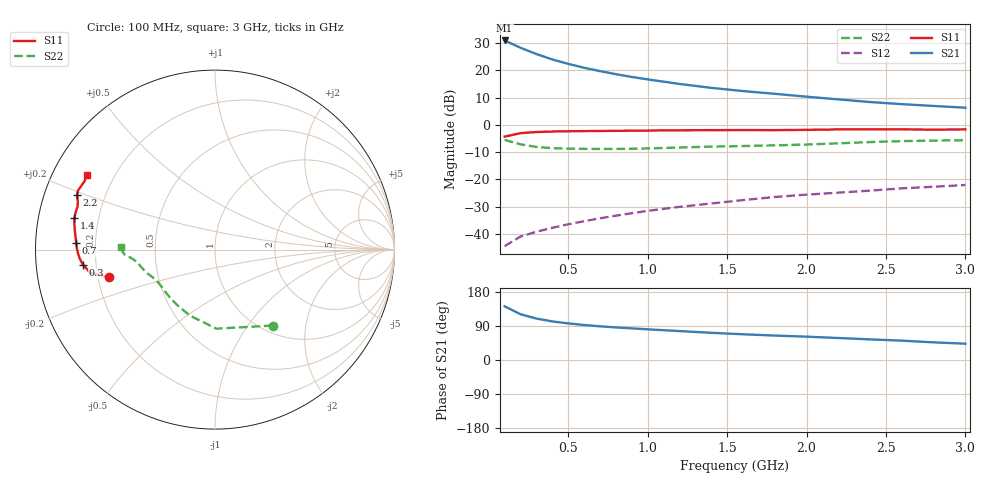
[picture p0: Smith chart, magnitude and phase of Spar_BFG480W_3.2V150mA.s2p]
! Filename: 3_2150BFG480.001
! Title: BFG480W
! Bias: Vce=3.2V; Ic=150mA
! Company: NXP Semiconductors NL
! User: Quality&Reliability T&D
! Measure time: 10 Nov 1999 / 11:58:59
#  MHz  S  MA  R 50
! Freq  S11  S21  S12  S22  :
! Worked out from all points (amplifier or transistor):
!   20 points, 100 MHz to 3 GHz, reference 50 ohm
!   highest |S21| = 30.9 dB at 100 MHz (marker M1)
!   |S21| within 3 dB of that: start of sweep to 213.9 MHz
!   unconditionally stable (mu >= 1): start of sweep to 121.3 MHz; 303.4 MHz to end of sweep
!   at 400 MHz: K = 1.07, MAG = 29.3 dB, |S12| = -37.7 dB
!   at 1.2 GHz: K = 1.20, MAG = 19.8 dB, |S12| = -30.0 dB
!   at 3 GHz: K = 1.16, MAG = 11.8 dB, |S12| = -22.0 dB
!   S11 on the Smith chart (normalised r, x): 100 MHz: 0.25, -0.12; 300 MHz: 0.15, -0.06; 700 MHz: 0.13, +0.02; 1.4 GHz: 0.11, +0.11; 2.2 GHz: 0.10, +0.19; 3 GHz: 0.10, +0.27
100  0.61 -165.3  35.22 141.7  0.006005 64.7  0.5311 -52.8
200  0.706 -169.4  25.87 120.8  0.008999 58.7  0.4406 -88.9
300  0.7401 -173.4  19.85 109.4  0.01103 60.2  0.3942 -110.2
400  0.756 -176.3  15.82 101.9  0.01303 63.0  0.3751 -123.4
500  0.7647 -178.8  13.13 96.5  0.01513 65.5  0.3674 -132.2
600  0.7703 179.2  11.13 92.3  0.01723 67.7  0.3639 -138.3
700  0.774 177.3  9.673 88.9  0.01948 70.0  0.3624 -142.9
800  0.7779 175.6  8.502 86.0  0.02173 71.5  0.3629 -146.7
900  0.7826 174.0  7.562 83.4  0.02411 73.3  0.3654 -149.9
1000  0.7877 172.4  6.818 81.0  0.02663 74.2  0.3704 -152.8
1200  0.7964 169.7  5.635 76.4  0.03151 75.4  0.3847 -157.3
1400  0.8021 167.5  4.77 71.8  0.03632 76.0  0.3998 -160.7
1600  0.8041 165.1  4.167 67.9  0.0419 76.6  0.4102 -163.5
1800  0.8021 162.6  3.711 64.5  0.04782 76.8  0.4217 -166.6
2000  0.8107 160.5  3.288 61.6  0.0528 77.3  0.4373 -170.4
2200  0.8266 158.5  2.933 58.1  0.05739 77.0  0.4596 -173.4
2400  0.8311 156.7  2.625 54.4  0.06248 76.3  0.4846 -175.5
2600  0.8262 154.8  2.398 51.0  0.06886 75.4  0.5043 -176.9
2800  0.8208 152.4  2.223 46.6  0.07362 73.9  0.5152 -178.6
3000  0.8251 149.7  2.064 43.1  0.07913 73.0  0.525 178.6
